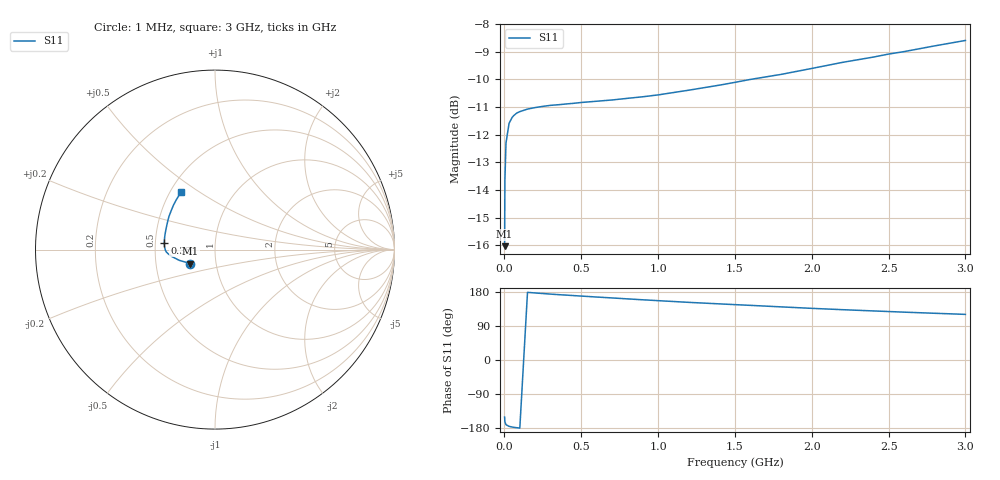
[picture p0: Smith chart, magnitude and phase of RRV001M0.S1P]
! SIEMENS Small Signal Semiconductors
! BA595
! Si PIN Diode in SOD323
! IF = 1 mA
! S-Parameters:  July  1992
# GHz  S  MA  R  50
!  f  S11
! GHz  MAG  ANG
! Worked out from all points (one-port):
!   33 points, 1 MHz to 3 GHz, reference 50 ohm
!   lowest |S11| = -16.0 dB at 1 MHz (marker M1), VSWR 1.38, Z = 37.5 - j5.97 ohm
!   |S11| at or under -10 dB: start of sweep to 1.601 GHz
!   S11 on the Smith chart (normalised r, x): 1 MHz: 0.75, -0.12; 350 MHz: 0.56, +0.05; 3 GHz: 0.57, +0.42
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0.001  0.158 -150.6
0.003  0.208 -163.3
0.01  0.2427 -170.7
0.03  0.2634 -175.1
0.05  0.27 -176.9
0.06  0.272 -177.5
0.08  0.2749 -178.7
0.1  0.2766 -179.6
0.15  0.2795 178.5
0.2  0.2813 176.9
0.3  0.2839 173.9
0.35  0.2846 172.5
0.4  0.2855 171.3
0.5  0.2873 168.7
0.6  0.2888 166.2
0.8  0.2923 161.3
1  0.2965 156.6
1.2  0.3024 152.1
1.4  0.3088 148.1
1.6  0.3162 144.2
1.8  0.3229 140.2
2  0.331 136.3
2.2  0.3395 132.8
2.4  0.347 129.5
2.5  0.3514 127.9
2.6  0.355 126.3
2.8  0.3636 123.3
3  0.3719 120.4
